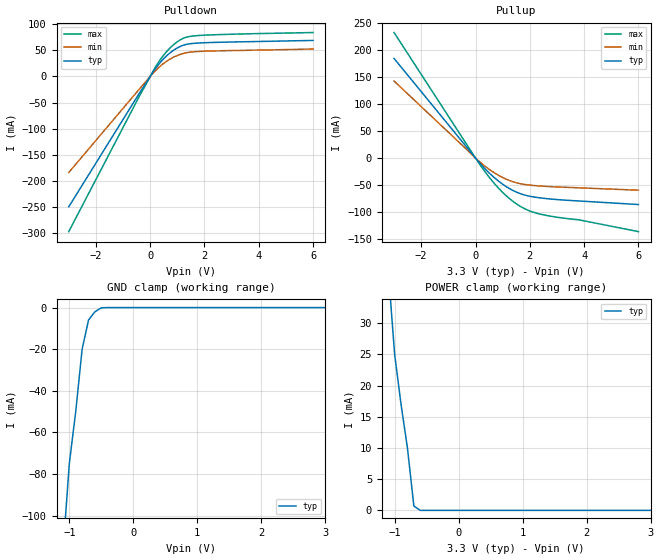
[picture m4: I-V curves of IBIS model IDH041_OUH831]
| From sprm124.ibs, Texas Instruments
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[Model]   IDH041_OUH831
Model_type   I/O
Polarity   Non-Inverting
Enable   Active-Low
| signals
Vinl = 0.8V
Vinh = 2.0V
Cref = 30p
Rref = 50
Vref = 1.5
Vmeas = 1.5
|   typ   min   max
C_comp   4.2150p   4.1750p   4.6940p
|   typ   min   max
[Temperature Range]   25.0   0   90
|   typ   min   max
[Voltage Range]   3.3V   3.13V   3.47V
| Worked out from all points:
|   slope of the pulldown table from 0 to 0.495 V, typ, clamps not added: 14.6 ohm
|   slope of the pullup table from 0 to 0.495 V, typ, clamps not added: 18.2 ohm
|   GND clamp passes 1 mA (typ) near -0.55 V on its own axis
|   POWER clamp passes 1 mA (typ) near -0.70 V on its own axis
[Pulldown]
|   Voltage   I(typ)   I(min)   I(max)
-3V       -249.9mA   -184.2mA   -297.4mA
-400mV    -32.25mA   -24.28mA   -37.96mA
100mV     8.09mA     5.916mA    9.684mA
300mV     22.32mA    16.37mA    26.78mA
500mV     34.16mA    25.1mA     41.09mA
900mV     51.51mA    37.89mA    62.44mA
1.1V      57.32mA    42.16mA    69.83mA
1.3V      61.06mA    45.09mA    74.68mA
1.7V      63.76mA    47.59mA    78.07mA
6V        68.96mA    52.46mA    84.1mA
[GND_clamp]
|   Voltage   I(typ)   I(min)   I(max)
-3V       -900mA     NA         NA
-2V       -500mA     NA         NA
-1V       -75mA      NA         NA
-900mV    -50mA      NA         NA
-800mV    -20mA      NA         NA
-700mV    -6mA       NA         NA
-600mV    -2mA       NA         NA
-500mV    -120uA     NA         NA
-400mV    0A         NA         NA
3V        0A         NA         NA
[Pullup]
|   Voltage   I(typ)   I(min)   I(max)
-3V       184.5mA    142.7mA    232.5mA
200mV     -11.72mA   -8.99mA    -14.95mA
500mV     -27.42mA   -20.82mA   -35.32mA
800mV     -40.84mA   -30.65mA   -53.18mA
1.3V      -57.99mA   -42.58mA   -77.18mA
1.8V      -68.47mA   -48.95mA   -93.68mA
2.3V      -73.3mA    -51.54mA   -102.9mA
3V        -76.95mA   -53.6mA    -109.7mA
3.8V      -79.56mA   -55.19mA   -114.4mA
6V        -86.16mA   -59.59mA   -136.4mA
[POWER_clamp]
|   Voltage   I(typ)   I(min)   I(max)
-3V       300mA      NA         NA
-2V       160mA      NA         NA
-1V       25mA       NA         NA
-900mV    17mA       NA         NA
-800mV    10mA       NA         NA
-700mV    700uA      NA         NA
-600mV    0A         NA         NA
-500mV    0A         NA         NA
3V        0A         NA         NA
[Ramp]
|   I(typ)   I(min)   I(max)
dV/dt_r   1.478/0.190n   1.242/0.240n   1.641/0.160n
dV/dt_f   1.406/0.200n   1.188/0.250n   1.600/0.160n
